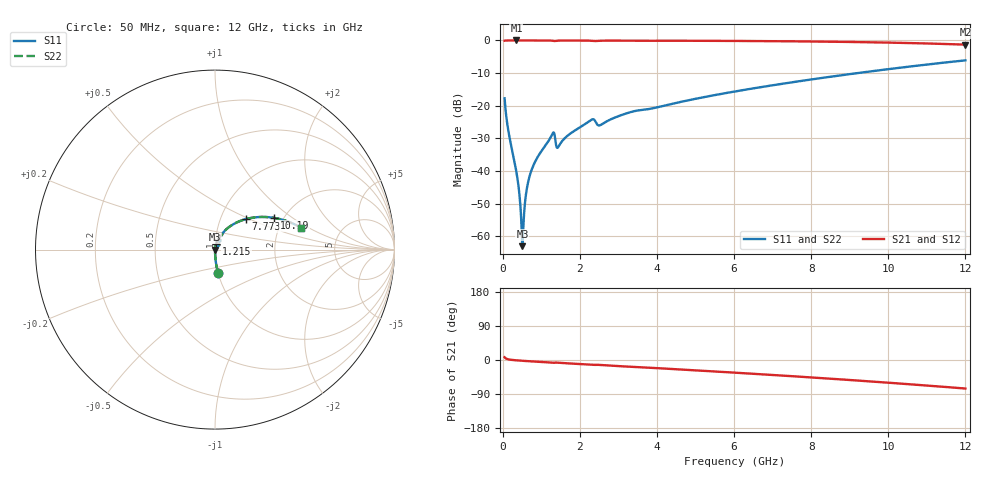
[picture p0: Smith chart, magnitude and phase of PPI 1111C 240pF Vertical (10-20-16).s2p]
# GHz S MA R 50
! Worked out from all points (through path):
!   1601 points, 50 MHz to 12 GHz, reference 50 ohm
!   highest |S21| = -0.01 dB at 356.2 MHz (marker M1); lowest = -1.3 dB at 12 GHz (marker M2)
!   group delay of S21, straight-line fit = 17.3 ps
!   lowest |S11| = -63.0 dB at 513.1 MHz (marker M3), VSWR 1.00, Z = 50.1 + j0.000529 ohm
!   |S11| at or under -10 dB: start of sweep to 9.201 GHz
!   |S22| runs from -63.0 to -6.1 dB; largest |S21 - S12| = 0
!   S11 on the Smith chart (normalised r, x): 50 MHz: 1.00, -0.26; 1.215 GHz: 1.01, +0.06; 7.773 GHz: 1.32, +0.47; 10.19 GHz: 1.79, +0.74; 12 GHz: 2.65, +0.85
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0.05  0.13 -82.6  0.9912 7.3  0.9912 7.3  0.13 -82.6
0.1620312  0.03678 -87.9  0.9989 1.5  0.9989 1.5  0.03678 -87.9
0.3562187  0.00967 -87.3  0.9993 -0.9  0.9993 -0.9  0.00967 -87.3
0.4159687  0.005505 -84.6  0.9993 -1.4  0.9993 -1.4  0.005505 -84.6
0.4757188  0.002059 -72.4  0.9993 -1.8  0.9993 -1.8  0.002059 -72.4
0.5130625  0.0007082 0.4  0.9993 -2.1  0.9993 -2.1  0.0007082 0.4
0.5504062  0.00201 66.3  0.9992 -2.3  0.9992 -2.3  0.00201 66.3
0.6325625  0.005639 79.2  0.9992 -2.9  0.9992 -2.9  0.005639 79.2
0.7296563  0.009613 81.5  0.9991 -3.5  0.9991 -3.5  0.009613 81.5
1.215125  0.03068 77.6  0.9964 -6.7  0.9964 -6.7  0.03068 77.6
1.30475  0.03861 64.8  0.9874 -7.4  0.9874 -7.4  0.03861 64.8
1.446656  0.02362 67.8  0.9935 -7.2  0.9935 -7.2  0.02362 67.8
2.044156  0.04841 76.0  0.9962 -11.0  0.9962 -11.0  0.04841 76.0
2.313031  0.06171 67.1  0.9872 -12.8  0.9872 -12.8  0.06171 67.1
2.522156  0.05024 65.7  0.9888 -13.0  0.9888 -13.0  0.05024 65.7
4.038312  0.09549 64.8  0.9893 -21.7  0.9893 -21.7  0.09549 64.8
6.025  0.1655 55.5  0.9826 -33.4  0.9826 -33.4  0.1655 55.5
7.772687  0.2414 44.7  0.9665 -44.5  0.9665 -44.5  0.2414 44.7
8.019156  0.2534 43.1  0.9633 -46.1  0.9633 -46.1  0.2534 43.1
10.01331  0.3642 29.3  0.9265 -60.0  0.9265 -60.0  0.3642 29.3
10.18509  0.3748 28.1  0.9222 -61.3  0.9222 -61.3  0.3748 28.1
12  0.4957 14.2  0.8627 -75.3  0.8627 -75.3  0.4957 14.2
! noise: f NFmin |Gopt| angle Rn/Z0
0.05  0.0003685  0.8648  0.2822  0.0005853
1.372  0.01512  0.9077  5.549  0.03588
2.701  0.01059  0.7615  10.77  0.008925
4.031  0.01503  0.7527  15.94  0.01203
5.36  0.01296  0.6461  20.56  0.006731
6.682  0.01453  0.6186  25.07  0.006781
8.012  0.01665  0.6101  29.49  0.00743
9.341  0.01907  0.6113  33.76  0.00838
10.67  0.02183  0.6194  37.91  0.009626
12  0.02498  0.6331  41.95  0.01124
